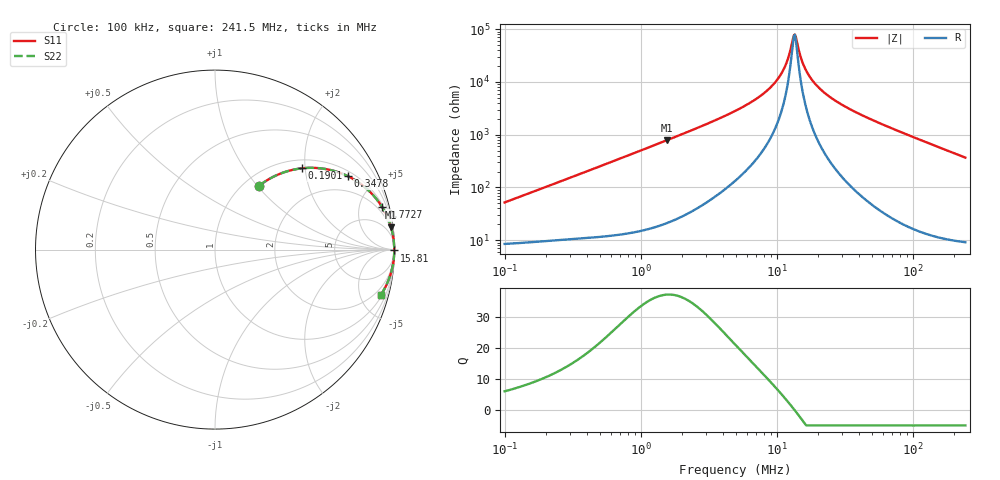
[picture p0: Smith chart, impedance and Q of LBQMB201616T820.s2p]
! LBQMB201616T820  S-PARAMETER MODEL  ( General Type )
! Model Generated by TAIYO YUDEN Corporation (http://www.ty-top.com)
! Version 1.0
! TAIYO YUDEN Control No. 191025NI43SB-FBB
! Copyright(c) 2019 TAIYO YUDEN CO.,LTD. All Rights Reserved.
! Product Description (link to TY-COMPAS)
! https://ds.yuden.co.jp/TYCOMPAS/or/detail?pn=LBQMB201616T820J&u=M
! Products Name : Inductors
! Characteristics :
!  Inductance : 82 uH , SRF(min) : 10 MHz , DC Resistance(max) : 10.01 Ohm , Rated Current : 85 mA
!  Case Size : 2.0 x 1.6 / 0.079 x 0.063 [mm/inch] , Thickness : 1.6 / 0.063 [mm/inch]
!  (Conditions: Temperature = 25 degC , DC Bias Current/Voltage = 0A / 0V)
! External Node Assignments :
!  1  o---GGG---o  2
! GND o---------o GND
! Frequency Range : 0.1MHz  -  241.513628MHz  [ 402 STEP ]
# MHz S RI R 50
! Freq[MHz].  S11 Real  S11 Imag  S21 Real  S21 Imag  S12 Real  S12 Imag  S22 Real  S22 Imag
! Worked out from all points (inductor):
!   401 points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, 100 kHz to 241.5 MHz, reference 50 ohm
!   read as one part in series: L = 81.1 uH near 104 kHz
!   highest Q = 37.3 at 1.558 MHz (marker M1), where L = 80.3 uH
!   self-resonance near 13.27 MHz
!   S11 on the Smith chart (normalised r, x): 100 kHz: 1.17, +1.02; 190.1 kHz: 1.19, +1.93; 347.8 kHz: 1.21, +3.49; 772.7 kHz: 1.26, +7.74; 15.81 MHz: open; 241.5 MHz: 1.18, -7.34
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0.1  0.2456 0.3555  0.7544 -0.3555  0.7544 -0.3555  0.2456 0.3555
0.190148  0.4849 0.453  0.5151 -0.453  0.5151 -0.453  0.4849 0.453
0.347753  0.741 0.4086  0.259 -0.4086  0.259 -0.4086  0.741 0.4086
0.368674  0.7618 0.3979  0.2382 -0.3979  0.2382 -0.3979  0.7618 0.3979
0.77272  0.9303 0.2382  0.0697 -0.2382  0.0697 -0.2382  0.9303 0.2382
1.359207  0.9754 0.1419  0.0246 -0.1419  0.0246 -0.1419  0.9754 0.1419
1.557711  0.9809 0.1243  0.0191 -0.1243  0.0191 -0.1243  0.9809 0.1243
4.914404  0.9971 0.0354  0.00293 -0.0354  0.00293 -0.0354  0.9971 0.0354
7.397334  0.9982 0.019  0.00183 -0.019  0.00183 -0.019  0.9982 0.019
9.715792  0.9985 0.00996  0.00145 -0.00996  0.00145 -0.00996  0.9985 0.00996
10.7094  0.9986 0.00692  0.00136 -0.00692  0.00136 -0.00692  0.9986 0.00692
11.57696  0.9987 0.00454  0.00131 -0.00454  0.00131 -0.00454  0.9987 0.00454
13.01183  0.9987 0.001  0.00125 -0.001  0.00125 -0.001  0.9987 0.001
13.26771  0.9988 0.000415  0.00125 -0.000415  0.00125 -0.000415  0.9988 0.000415
13.79465  0.9988 -0.00076  0.00124 0.00076  0.00124 0.00076  0.9988 -0.00076
14.91214  0.9988 -0.00312  0.00123 0.00312  0.00123 0.00312  0.9988 -0.00312
15.80928  0.9988 -0.0049  0.00123 0.0049  0.00123 0.0049  0.9988 -0.0049
18.11814  0.9987 -0.00914  0.00126 0.00914  0.00126 0.00914  0.9987 -0.00914
22.0134  0.9986 -0.0155  0.00139 0.0155  0.00139 0.0155  0.9986 -0.0155
28.3552  0.9982 -0.0247  0.00176 0.0247  0.00176 0.0247  0.9982 -0.0247
66.79689  0.9933 -0.0719  0.00665 0.0719  0.00665 0.0719  0.9933 -0.0719
241.5136  0.9257 -0.2502  0.0743 0.2502  0.0743 0.2502  0.9257 -0.2502
